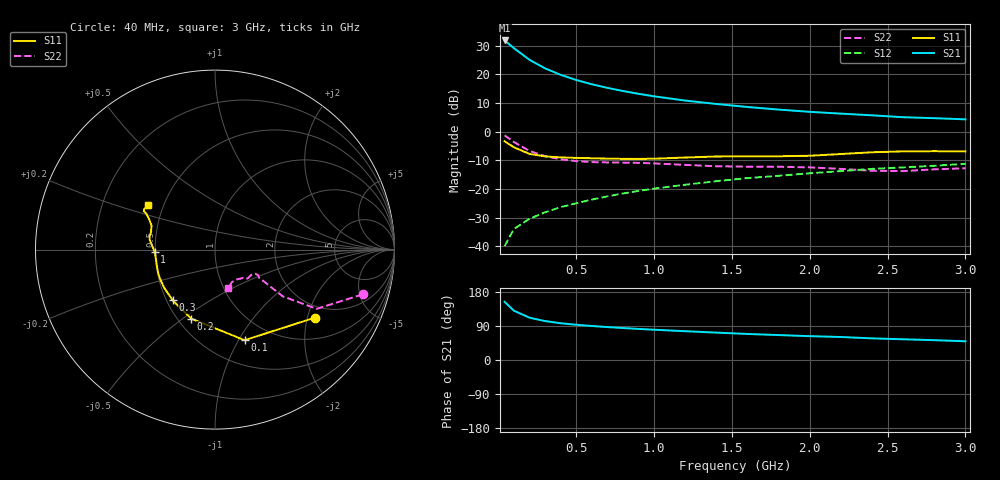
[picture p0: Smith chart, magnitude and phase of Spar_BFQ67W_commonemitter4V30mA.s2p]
! Filename:  BFQ67WF.S2P  Version:  4.0
! NXP part #: BFQ67W  Date: Jun 1994
! Bias condition: Vce=4V, Ic=30mA
#  MHz  S  MA  R  50
! Freq  S11  S21  S12  S22  !GUM [dB]
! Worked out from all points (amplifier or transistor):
!   21 points, 40 MHz to 3 GHz, reference 50 ohm
!   highest |S21| = 31.8 dB at 40 MHz (marker M1)
!   |S21| within 3 dB of that: start of sweep to 107.4 MHz
!   unconditionally stable (mu >= 1): 469.9 MHz to 2.989 GHz
!   at 300 MHz: K = 0.88, MSG = 25.1 dB, |S12| = -28.2 dB
!   at 1 GHz: K = 1.10, MAG = 14.2 dB, |S12| = -19.9 dB
!   at 3 GHz: K = 1.00, MSG = 7.8 dB, |S12| = -11.3 dB
!   lowest NFmin = 2.50 dB at 1 GHz
!   S11 on the Smith chart (normalised r, x): 40 MHz: 1.61, -2.24; 100 MHz: 0.75, -1.06; 200 MHz: 0.58, -0.54; 300 MHz: 0.54, -0.35; 1 GHz: 0.50, -0.02; 3 GHz: 0.41, +0.26
40  0.675 -34.1  38.83 153.5  0.01 75.5  0.859 -16.9
100  0.531 -71.9  28.46 130.0  0.02 63.5  0.656 -30.2
200  0.407 -109.0  17.81 111.6  0.03 61.6  0.459 -34.6
300  0.368 -129.9  12.66 102.7  0.039 63.8  0.372 -33.8
400  0.354 -143.1  9.753 97.0  0.048 66.6  0.328 -33.1
500  0.347 -151.6  7.93 93.0  0.056 68.6  0.305 -32.8
600  0.342 -158.0  6.683 89.7  0.065 70.1  0.293 -32.7
700  0.337 -163.5  5.784 86.9  0.074 71.4  0.289 -32.4
800  0.334 -168.4  5.096 84.4  0.083 72.3  0.287 -31.8
900  0.333 -173.1  4.559 82.0  0.092 72.9  0.284 -31.2
1000  0.336 -177.5  4.117 79.9  0.101 73.3  0.278 -30.7
1200  0.352 176.0  3.471 76.0  0.118 73.8  0.262 -30.9
1400  0.367 171.9  3.027 72.3  0.136 74.3  0.248 -33.9
1600  0.371 168.6  2.681 68.7  0.154 73.7  0.244 -38.6
1800  0.37 164.5  2.416 65.8  0.169 73.9  0.243 -41.5
2000  0.378 159.3  2.208 62.9  0.187 74.0  0.237 -42.7
2200  0.405 155.1  2.053 60.7  0.204 74.3  0.223 -45.2
2400  0.435 152.2  1.919 57.1  0.223 73.7  0.207 -52.9
2600  0.451 151.7  1.778 54.7  0.237 73.0  0.204 -62.6
2800  0.454 150.3  1.711 52.3  0.253 73.1  0.219 -68.3
3000  0.451 146.2  1.632 49.4  0.273 72.5  0.229 -71.0
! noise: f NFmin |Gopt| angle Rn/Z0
1000  2.5  0.158  140  0.323
